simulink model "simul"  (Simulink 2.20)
settings: Solver=ode45  StartTime=0.0  StopTime=100.0  RelTol=1e-3  AbsTol=1e-6
libraries: simulink x2

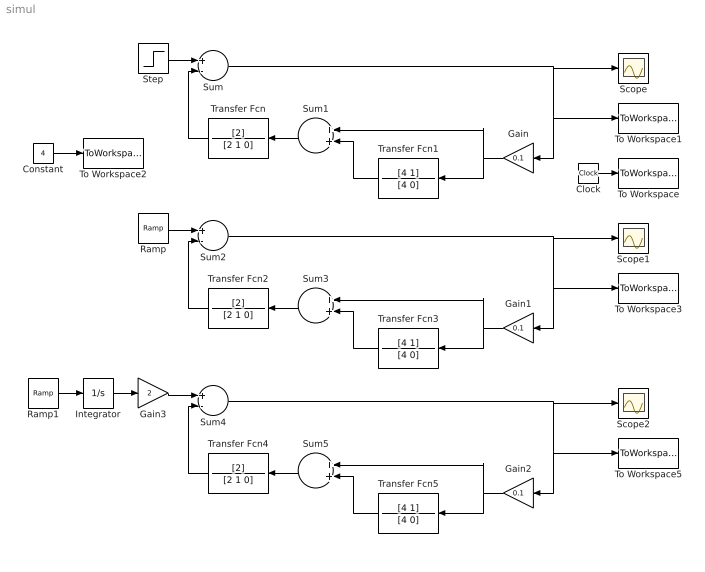
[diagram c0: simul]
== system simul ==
  Clock : Clock
  Constant : Constant  Value=4
  Gain : Gain  Orientation=left  Gain=0.1
  Gain1 : Gain  Orientation=left  Gain=0.1
  Gain2 : Gain  Orientation=left  Gain=0.1
  Gain3 : Gain  Gain=2
  Integrator : Integrator  ExternalReset=none  InitialConditionSource=internal  InitialCondition=0  LimitOutput=off  UpperSaturationLimit=inf  LowerSaturationLimit=-inf  ShowSaturationPort=off  ShowStatePort=off  AbsoluteTolerance=auto
  Ramp : simulink/Sources/Ramp  slope=1  start=0  X0=0
  Ramp1 : simulink/Sources/Ramp  slope=1  start=0  X0=0
  Scope : Scope
  Scope1 : Scope
  Scope2 : Scope
  Step : Step  Time=0  Before=0  After=1
  Sum : Sum  Inputs=+-
  Sum1 : Sum  Orientation=left  Inputs=++
  Sum2 : Sum  Inputs=+-
  Sum3 : Sum  Orientation=left  Inputs=++
  Sum4 : Sum  Inputs=+-
  Sum5 : Sum  Orientation=left  Inputs=++
  To Workspace : ToWorkspace  VariableName=clocksim  SampleTime=-1
  To Workspace1 : ToWorkspace  VariableName=stepsim  SampleTime=-1
  To Workspace2 : ToWorkspace  VariableName=k  SampleTime=-1
  To Workspace3 : ToWorkspace  VariableName=rampsim  SampleTime=-1
  To Workspace5 : ToWorkspace  VariableName=sqsim  SampleTime=-1
  Transfer Fcn : TransferFcn  Orientation=left  Numerator=[2]  Denominator=[2 1 0]
  Transfer Fcn1 : TransferFcn  Orientation=left  Numerator=[4 1]  Denominator=[4 0]
  Transfer Fcn2 : TransferFcn  Orientation=left  Numerator=[2]  Denominator=[2 1 0]
  Transfer Fcn3 : TransferFcn  Orientation=left  Numerator=[4 1]  Denominator=[4 0]
  Transfer Fcn4 : TransferFcn  Orientation=left  Numerator=[2]  Denominator=[2 1 0]
  Transfer Fcn5 : TransferFcn  Orientation=left  Numerator=[4 1]  Denominator=[4 0]
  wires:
  Step/1 -> Sum/1
  Transfer Fcn/1 -> Sum/2
  Transfer Fcn1/1 -> Sum1/2
  Gain/1 -> Transfer Fcn1/1, Sum1/1
  Sum/1 -> Scope/1, To Workspace1/1, Gain/1
  Clock/1 -> To Workspace/1
  Ramp/1 -> Sum2/1
  Transfer Fcn2/1 -> Sum2/2
  Transfer Fcn3/1 -> Sum3/2
  Gain1/1 -> Transfer Fcn3/1, Sum3/1
  Sum2/1 -> Gain1/1, To Workspace3/1, Scope1/1
  Gain3/1 -> Sum4/1
  Transfer Fcn4/1 -> Sum4/2
  Transfer Fcn5/1 -> Sum5/2
  Gain2/1 -> Transfer Fcn5/1, Sum5/1
  Sum4/1 -> Scope2/1, To Workspace5/1, Gain2/1
  Integrator/1 -> Gain3/1
  Ramp1/1 -> Integrator/1
  Sum1/1 -> Transfer Fcn/1
  Sum3/1 -> Transfer Fcn2/1
  Sum5/1 -> Transfer Fcn4/1
  Constant/1 -> To Workspace2/1
